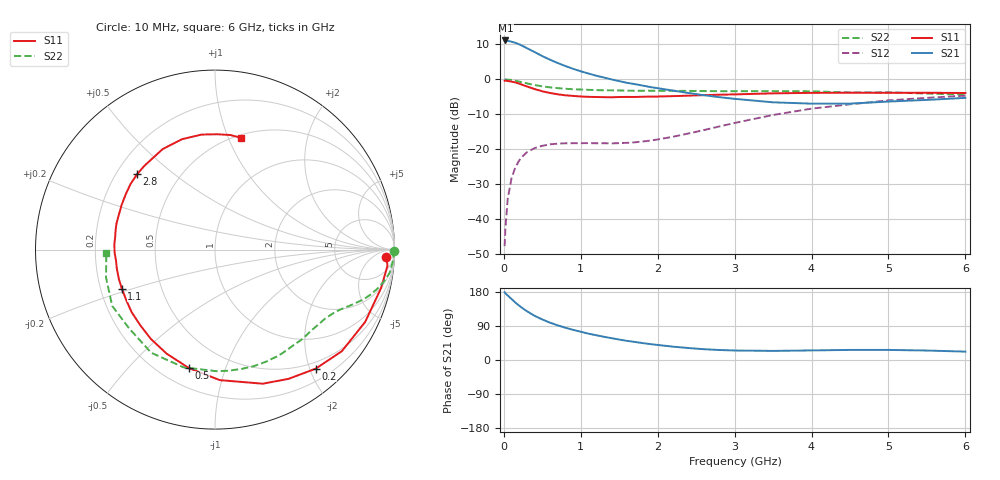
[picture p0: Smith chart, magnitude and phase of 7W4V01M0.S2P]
! Infineon Technologies  Discrete & RF Semiconductors
! BFS17W
! Si NPN RF Bipolar Junction Transistor in SOT323
! VCE = 4 V  IC = 1 mA
! Common Emitter S-Parameters:  August  1999
# GHz  S  MA  R  50
!  f  S11  S21  S12  S22
! GHz  MAG  ANG  MAG  ANG  MAG  ANG  MAG  ANG
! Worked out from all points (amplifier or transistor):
!   36 points, 10 MHz to 6 GHz, reference 50 ohm
!   highest |S21| = 11.2 dB at 20 MHz (marker M1)
!   |S21| within 3 dB of that: start of sweep to 371 MHz
!   unconditionally stable (mu >= 1): 1.046 GHz to end of sweep
!   at 250 MHz: K = 0.26, MSG = 15.7 dB, |S12| = -21.9 dB
!   at 1.4 GHz: K = 1.27, MAG = 6.0 dB, |S12| = -18.3 dB
!   at 6 GHz: K = 1.10, MAG = -2.2 dB, |S12| = -4.7 dB
!   S11 on the Smith chart (normalised r, x): 10 MHz: 23, -22; 200 MHz: 0.39, -2.10; 500 MHz: 0.31, -0.76; 1.1 GHz: 0.29, -0.18; 2.8 GHz: 0.28, +0.38; 6 GHz: 0.53, +1.11
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0.01  0.9564 -2.5  3.585 178.8  0.0041 87.3  0.9999 -0.3
0.02  0.9652 -5.4  3.611 176.2  0.0073 89.1  0.9955 -1.5
0.05  0.9496 -13.1  3.571 170.2  0.0194 84.2  0.9931 -3.9
0.1  0.9288 -25.7  3.466 161.0  0.0386 75.2  0.9815 -7.6
0.15  0.9055 -38.7  3.341 151.6  0.0551 67.9  0.9558 -10.9
0.2  0.8687 -49.8  3.184 143.3  0.0694 62.5  0.9302 -13.6
0.25  0.8284 -60.4  2.99 135.7  0.0806 56.5  0.9024 -16.1
0.3  0.7931 -70.4  2.803 128.8  0.0906 52.3  0.8781 -18.1
0.4  0.7277 -87.9  2.462 116.6  0.104 44.8  0.8307 -21.4
0.5  0.676 -102.4  2.156 107.0  0.112 39.6  0.7964 -23.8
0.6  0.6391 -115.0  1.914 98.5  0.1176 36.1  0.7698 -25.9
0.7  0.6127 -125.7  1.717 91.5  0.1204 34.0  0.7506 -28.0
0.9  0.5807 -143.1  1.418 79.6  0.1221 31.4  0.7235 -32.2
1.1  0.5629 -157.3  1.214 69.5  0.1225 32.0  0.7089 -36.7
1.6  0.5614 176.6  0.894 50.5  0.1235 40.7  0.6908 -49.1
2.2  0.5764 154.6  0.691 35.2  0.1512 56.6  0.686 -65.9
2.8  0.6037 136.0  0.557 26.4  0.212 64.3  0.679 -83.8
3.5  0.6315 117.5  0.47 24.0  0.3097 62.9  0.679 -104.9
4.5  0.6452 96.7  0.45 26.6  0.4401 50.6  0.6494 -137.3
5  0.6428 89.0  0.482 26.6  0.5011 44.0  0.6529 -151.2
5.5  0.6441 82.3  0.509 25.0  0.5449 37.3  0.6268 -165.6
6  0.6391 77.1  0.544 22.1  0.5853 31.0  0.6059 -178.1
